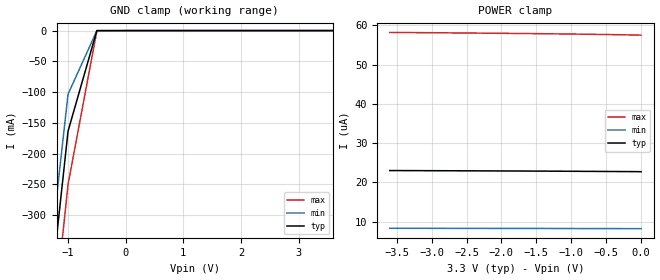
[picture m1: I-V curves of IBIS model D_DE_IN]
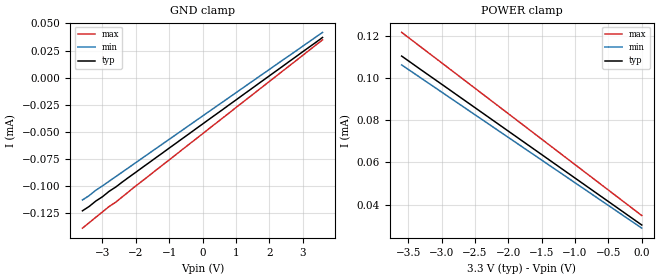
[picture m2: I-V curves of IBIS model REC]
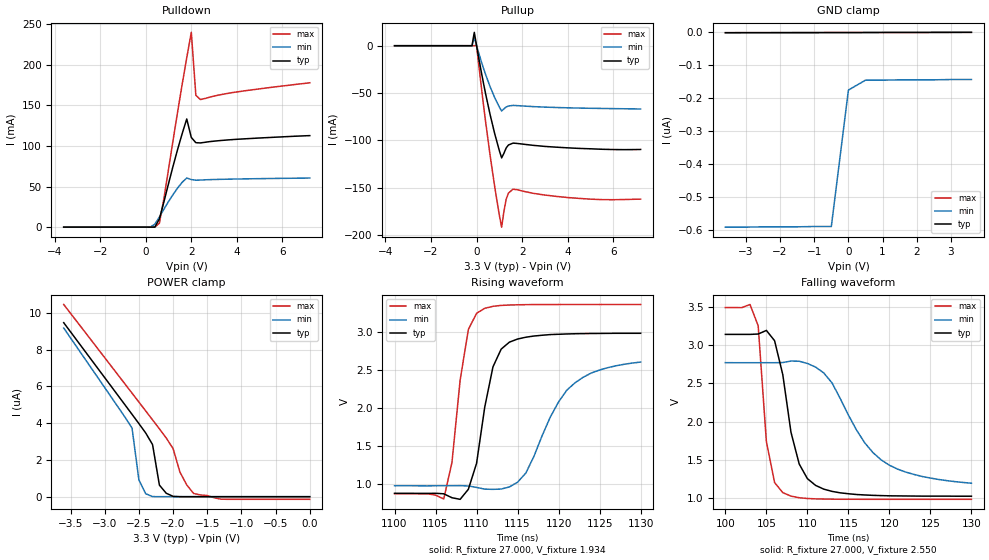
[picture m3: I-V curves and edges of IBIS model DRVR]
|   Texas Instruments Incorporated
|   Data Transmissions Products
|   IBIS Model for SN65HVD79
|   8D SOIC Package
[IBIS Ver]   3.2
[Comment char]   |_char
[File name]   hvd379.ibs
[File Rev]   1.0
[Date]   29Mar07
[Source]   File originated at Texas Instruments Incorporated.
   Data Transmission Products Group.
[Notes]
[Disclaimer]
(C) Copyright Texas Instruments Incorporated 2002
   All rights reserved
  Texas Instruments Incorporated hereby grants the user of this IBIS
model a non-exclusive, nontransferable license to use this IBIS model
under the following terms.  Before using this IBIS model, the user
should read this license.  If the user does not accept these terms,
the IBIS model should be returned to Texas Instruments within 30 days.
  The user is granted this license only to use the IBIS model and
is not granted rights to sell, load, rent, lease or license the IBIS
model in whole or in part, or in modified form to anyone other than
user.  User may modify the IBIS model to suit its specific applications
but rights to derivative works and such modifications shall belong to
Texas Instruments.
  This IBIS model is provided on an "AS IS" basis and Texas Instruments
makes absolutely no warranty with respect to the information contained
herein.  TEXAS INSTRUMENTS DISCLAIMS AND CUSTOMER WAIVES ALL WARRANTIES,
EXPRESS OR IMPLIED, INCLUDING WARRANTIES OF MERCHANTABILITY OR FITNESS
FOR A PARTICULAR PURPOSE. The entire risk as to quality and performance
is with the Customer. ACCORDINGLY, IN NO EVENT SHALL THE COMPANY BE LIABLE
FOR ANY DAMAGES, WHETHER IN CONTRACT OR TORT,INCLUDING ANY LOST PROFITS
OR OTHER INCIDENTAL, CONSEQUENTIAL, EXEMPLARY, OR PUNITIVE DAMAGES ARISING
OUT OF THE USE OR APPLICATION OF THE IBIS model provided in this package.
Further, Texas Instruments reserves the right to discontinue or make changes
without notice to any product herein to improve reliability, function, or
design. Texas Instruments does not convey any license under patent rights
or any other intellectual property rights, including those of third parties.
Contact Texas Instruments at ATTN:DATA TRANSMISSIONS
[Copyright]   Copyright 2002, Texas Instruments, All Rights Reserved
[Component]   HVD379D
[Manufacturer]  Texas Instruments Incorporated
[Package]
|   typ   min   max
R_pkg   0.071   0.050   0.091
L_pkg   2.203nH   1.540nH   2.930nH
C_pkg   0.465pF   0.385pF   0.609pF
[Pin]   signal_name   model_name   R_pin   L_pin   C_pin
1   VCC   POWER   0.091   2.615n   0.500p
2   R   RECEIVER_OUT   0.076   2.346n   0.483p
3   D   D_DE_IN   0.062   1.755n   0.395p
4   GND   GND   0.090   2.593n   0.498p
5   Y   DRVR   0.073   2.300n   0.480p
6   Z   DRVR   0.076   2.012n   0.407p
7   B   REC   0.050   1.540n   0.385p
8   A   REC   0.070   1.897n   0.412p
[Diff_pin]   inv_pin   vdiff   tdelay_typ   tdelay_min   tdelay_max
| The 'A' pin is Diff_pin and the 'B' pin is the inv_pin
5   6   0.200   0 0 0
7   8   0.200   0 0 0
| Models and submodels in the file (4): D_DE_IN (Input), REC (Input), DRVR (I/O), RECEIVER_OUT (Output)
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|   Driver Input / Driver Enable / Model
[Model]   D_DE_IN
Model_type   Input
|Signals   D
Vinh = 2.0
Vinl = 0.8
|   typ   min   max
C_comp   23pF   19pF   27pF
|   typ   min   max
[Temperature Range]   27   -40   85
[Voltage range]   3.3V   3.0V   3.6V
[GND_clamp]
|   Voltage   I(typ)   I(min)   I(max)
-3.6V     -2.348A    -2.232A    -2.506A
-1.5V     -596.3mA   -523.6mA   -696.4mA
-1V       -163.5mA   -103.3mA   -250mA
-500mV    -12.8uA    -27.56uA   -399.4uA
3.6V      22.76uA    57.48uA    8.245uA
[Power_clamp]
| Note that the[POWER_clamp]voltage table is referenced to Vcc
| and is calculated using Vtable=Vcc - Vmeasured.
|   Voltage   I(typ)   I(min)   I(max)
-3.6V     23.01uA    8.325uA    58.18uA
-3.5V     23.01uA    8.322uA    58.16uA
-3.1V     22.98uA    8.313uA    58.11uA
-2.8V     22.97uA    8.306uA    58.07uA
-2V       22.91uA    8.286uA    57.95uA
-1.7V     22.89uA    8.278uA    57.89uA
-1.6V     22.88uA    8.276uA    57.88uA
-1.4V     22.87uA    8.27uA     57.84uA
-900mV    22.82uA    8.255uA    57.74uA
-500mV    22.78uA    8.242uA    57.64uA
-100mV    22.74uA    8.227uA    57.52uA
0V        22.72uA    8.222uA    57.48uA
|   Receiver Input / Model
[Model]   REC
Model_type   Input
|Signals   A,B
Vinh = 2.0
Vinl = 0.8
|   typ   min   max
C_comp   3pF   2.5pF   3.5pF
|   typ   min   max
[Temperature Range]   27   -40   85
[Voltage range]   3.3V   3.0V   3.6V
[GND_clamp]
|   Voltage   I(typ)   I(min)   I(max)
-3.6V     -123uA     -113uA     -139uA
-2.8V     -105uA     -95.7uA    -119uA
-2.6V     -101uA     -91.4uA    -115uA
3.6V      37.1uA     41.8uA     34.9uA
[Power_clamp]
| Note that the[POWER_clamp]voltage table is referenced to Vcc
| and is calculated using Vtable=Vcc - Vmeasured.
|   Voltage   I(typ)   I(min)   I(max)
-3.6V     110.3uA    106.1uA    121.5uA
-3.3V     103.6uA    99.69uA    114.3uA
-3V       96.98uA    93.26uA    107.1uA
-2.5V     85.89uA    82.54uA    95.07uA
-2V       74.79uA    71.82uA    83.04uA
-1.5V     63.7uA     61.1uA     71uA
-1V       52.6uA     50.38uA    58.96uA
-500mV    41.51uA    39.65uA    46.93uA
0V        30.41uA    28.93uA    34.89uA
|   Driver Output / Receiver Input Model
[Model]   DRVR
Model_type   I/O
| Signals   Y,Z
Vinl = 0.9V
Vinh = 2.8V
Vmeas = 1.7V   |Reference voltage for timing measurements
Cref = 50pF   |Timing specification test load capacitance value
Rref = 54   |Note: 54 Ohm load; single-ended configuration
|   Timing specification test load voltage
| variable   typ   min   max
C_comp   28pF   24pF   32pF
|   typ   min   max
[Temperature Range]   25.0   -40   85
[Voltage range]   3.3V   3.0V   3.6V
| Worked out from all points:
|   slope of the pulldown table from 0 to 0.495 V, typ, clamps not added: 101 ohm
|   slope of the pullup table from 0 to 0.495 V, typ, clamps not added: 7.99 ohm
|   rising waveform, R_fixture 27.000, V_fixture 1.934: 20-80 % time 2.05ns typ, 4.74ns min, 1.67ns max; typ from 0.872 V to 2.98 V
|   falling waveform, R_fixture 27.000, V_fixture 2.550: 20-80 % time 2.23ns typ, 5.64ns min, 1.3ns max; typ from 3.14 V to 1.03 V
[Pulldown]
|   Voltage   I(typ)   I(min)   I(max)
-3.6V     159.9pA    -3.538nA   187pA
200mV     102.5nA    84.16uA    637.5pA
400mV     125.5uA    3.658mA    2.583uA
600mV     10.13mA    12.54mA    4.944mA
800mV     31.32mA    22.18mA    35.61mA
1.2V      75.16mA    40.21mA    107mA
1.8V      133.2mA    60.51mA    208.6mA
2V        110.4mA    58.58mA    239.9mA
2.2V      104mA      57.81mA    162.4mA
2.4V      103.7mA    57.98mA    157.1mA
3.8V      107.8mA    59.18mA    165.7mA
7.2V      112.7mA    60.46mA    177.8mA
[Pullup]
|   Voltage   I(typ)   I(min)   I(max)
| Note that the[Pullup]voltage table is referenced to Vcc
| and is calculated using Vtable=Vcc - Vmeasured.
-3.6V     10.65uA    9.229uA    12.84uA
-200mV    2.036uA    2.463uA    2.347uA
-100mV    14.15mA    8.567mA    2.306uA
0V        206.6uA    144.9uA    382uA
300mV     -39.21mA   -23.56mA   -61.72mA
600mV     -73.39mA   -43.64mA   -116.8mA
1.1V      -118.5mA   -68.93mA   -191.7mA
1.3V      -108mA     -64.78mA   -162.1mA
1.4V      -104.9mA   -63.71mA   -155.7mA
1.6V      -102.9mA   -63.05mA   -151.6mA
4V        -107.9mA   -65.61mA   -160.4mA
7.2V      -109.6mA   -66.83mA   -162.1mA
[GND_clamp]
|   Voltage  I(typ)   I(min)   I(max)
| Outputs in High Impedance (off)
-3.6V     -974pA     -591nA     -897pA
-500mV    -651pA     -589nA     -575pA
0V        -527pA     -175nA     -523pA
500mV     -357pA     -145nA     -425pA
3.6V      186pA      -143nA     105pA
[POWER_clamp]
|   Voltage  I(typ)   I(min)   I(max)
| Note that the [POWER_clamp] voltage table is referenced to Vcc
| and is calculated using Vtable = Vcc - Vmeasured.
| Outputs in Tri-state.
-3.6V     9.461uA    9.171uA    10.45uA
-2.6V     4.476uA    3.728uA    5.628uA
-2.5V     3.975uA    913.7nA    5.145uA
-2.4V     3.462uA    159.9nA    4.662uA
-2.3V     2.832uA    5.888nA    4.177uA
-2.2V     629.7nA    839.3pA    3.69uA
-2.1V     188.2nA    418.3pA    3.19uA
-2V       18.21nA    442.3pA    2.618uA
-1.9V     1.35nA     417.4pA    1.34uA
-1.7V     446.8pA    389pA      176.4nA
-1.3V     361.5pA    326.9pA    -134nA
0V        132.8pA    105.2pA    -143.4nA
[Ramp]
|   typ   min   max
dV/dt_r   1.27V/3.8ns   0.96V/6.1ns   1.50V/1.7ns
dV/dt_f   1.27V/2.1ns   0.96V/4.7ns   1.50V/1.7ns
R_load = 27ohm | Note: The measurement is on a single-ended configuration
|   with 54ohm line-to-line.
[Rising Waveform]
R_fixture = 27.000
V_fixture = 1.934
V_fixture_min = 1.788
V_fixture_max = 2.122
C_fixture = 0.000
L_fixture = 0.000
|  time   V(typ)   V(min)   V(max)
1.1us     872mV      972.3mV    868mV
1.106us   866mV      972.3mV    798mV
1.107us   814mV      972.3mV    1.28V
1.108us   793mV      973.4mV    2.369V
1.109us   926mV      969.1mV    3.035V
1.11us    1.268V     950mV      3.249V
1.112us   2.542V     924.5mV    3.341V
1.114us   2.868V     956.4mV    3.358V
1.121us   2.976V     2.234V     3.365V
1.13us    2.985V     2.605V     3.365V
[Falling Waveform]
R_fixture = 27.000
V_fixture = 2.550
V_fixture_min = 2.276
V_fixture_max = 2.843
C_fixture = 0.000
L_fixture = 0.000
|  time   V(typ)   V(min)   V(max)
100ns     3.137V     2.769V     3.487V
103ns     3.137V     2.768V     3.527V
104ns     3.142V     2.768V     3.25V
105ns     3.189V     2.768V     1.739V
106ns     3.055V     2.768V     1.205V
107ns     2.612V     2.77V      1.074V
109ns     1.447V     2.787V     1.007V
111ns     1.168V     2.711V     992.2mV
119ns     1.035V     1.5V       986.2mV
130ns     1.027V     1.196V     986.2mV
